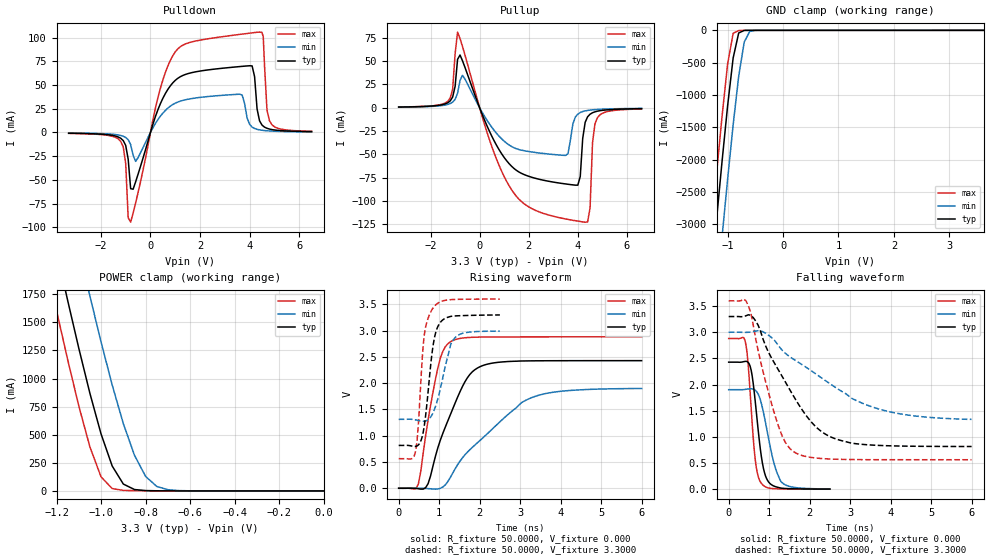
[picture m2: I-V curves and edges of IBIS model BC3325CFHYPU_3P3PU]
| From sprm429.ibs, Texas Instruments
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|   Model BC3325CFHYPU_3P3PU
[Model]   BC3325CFHYPU_3P3PU
Model_type   I/O
Polarity   Non-Inverting
Enable   Active-Low
Vinl =   0.9900V
Vinh =   2.3100V
Vmeas =   1.6500V
Cref =  15.0000pF
Rref = 100.0000M
Vref =  0.000V
C_comp   3.2113000062pf   3.3653001534pf   5.2276998132pf
[Temperature Range]   25.0000   0.1250k   -40.0000
[Voltage Range]   3.3000V   3.0000V   3.6000V
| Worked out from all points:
|   slope of the pulldown table from 0 to 0.495 V, typ, clamps not added: 13.9 ohm
|   slope of the pullup table from 0 to 0.495 V, typ, clamps not added: 16.3 ohm
|   GND clamp passes 1 mA (typ) near -0.67 V on its own axis
|   POWER clamp passes 1 mA (typ) near -0.73 V on its own axis
|   rising waveform, R_fixture 50.0000, V_fixture 0.000: 20-80 % time 712ps typ, 1.48ns min, 382ps max; typ from 0.001 V to 2.43 V
|   rising waveform, R_fixture 50.0000, V_fixture 3.3000: 20-80 % time 215ps typ, 312ps min, 166ps max; typ from 0.816 V to 3.3 V
|   falling waveform, R_fixture 50.0000, V_fixture 0.000: 20-80 % time 218ps typ, 319ps min, 166ps max; typ from 2.43 V to 0.003 V
|   falling waveform, R_fixture 50.0000, V_fixture 3.3000: 20-80 % time 1.13ns typ, 1.92ns min, 606ps max; typ from 3.3 V to 0.817 V
[Pulldown]
| voltage   I(typ)   I(min)   I(max)
-3.3V     -858uA     -614uA     -1.005mA
-1.2V     -6.162mA   -3.225mA   -9.462mA
-800mV    -59.28mA   -12.78mA   -94.65mA
-600mV    -52.16mA   -30.51mA   -74.44mA
1V        54.91mA    30.86mA    84.97mA
3.6V      69.44mA    40.27mA    103.4mA
4.1V      70.14mA    5.645mA    105mA
4.4V      12.22mA    2.696mA    105.8mA
4.55V     6.668mA    2.131mA    100.8mA
4.7V      4.353mA    1.744mA    23.59mA
4.8V      3.553mA    1.558mA    12.25mA
6.5V      840uA      548uA      1.176mA
|   6.6000   0.8040mA   0.5270mA   1.1160mA
[Pullup]
| voltage   I(typ)   I(min)   I(max)
-3.3V     805uA      687uA      859uA
-1.3V     5.391mA    3.609mA    6.959mA
-900mV    51.9mA     15.62mA    81.15mA
600mV     -35.88mA   -24.51mA   -49.07mA
1.7V      -70.21mA   -45.37mA   -100.4mA
3.5V      -81.59mA   -51.02mA   -119.1mA
4V        -82.9mA    -6.76mA    -121.4mA
4.3V      -15.54mA   -3.316mA   -122.6mA
4.5V      -6.855mA   -2.452mA   -107.1mA
4.6V      -5.294mA   -2.167mA   -37.4mA
4.8V      -3.613mA   -1.755mA   -10.57mA
6.6V      -914uA     -641uA     -1.25mA
[GND_clamp]
| voltage   I(typ)   I(min)   I(max)
-3.3V     -23.4A     -24.49A    -22.76A
-1.3V     -3.859A    -5.036A    -3.154A
-1.2V     -2.93A     -4.106A    -2.224A
-1.1V     -2.025A    -3.192A    -1.329A
-1V       -1.167A    -2.304A    -520.5mA
-900mV    -427.1mA   -1.461A    -46.43mA
-800mV    -40.98mA   -709.2mA   -2.872mA
-700mV    -1.416mA   -180.3mA   -459.5uA
-600mV    -185.8uA   -16.11mA   -224.9uA
-400mV    -135.4uA   -138.5uA   -210.3uA
3.62V     0A         0A         0A
[POWER_clamp]
| voltage   I(typ)   I(min)   I(max)
-3.3V     22.53A     23.34A     22.08A
-1.25V    2.586A     3.492A     2.054A
-1.2V     2.135A     3.04A      1.604A
-1.15V    1.695A     2.594A     1.168A
-1.05V    867.5mA    1.733A     390.4mA
-1V       506.6mA    1.325A     125mA
-950mV    221.5mA    942.3mA    21.03mA
-900mV    61.17mA    598.6mA    4.699mA
-850mV    12.39mA    317.4mA    2.279mA
-800mV    3.117mA    129.1mA    1.334mA
-750mV    1.236mA    39.97mA    732.8uA
0V        286.3pA    1.898nA    332.4pA
[Ramp]
| variable   typ   min   max
dV/dt_r   1.4399/0.6927n   0.7695/0.8573n   1.7265/0.3782n
dV/dt_f   1.3814/0.9941n   0.5983/0.9692n   1.8135/0.5956n
R_load = 50.0000
[Rising Waveform]
R_fixture = 50.0000
V_fixture = 0.000
V_fixture_min = 0.000
V_fixture_max = 0.000
| time   V(typ)   V(min)   V(max)
0s        1.182mV    1.135mV    1.272mV
484.8ps   -7.536mV   2.496mV    78.78mV
727.3ps   90.15mV    -4.991mV   1.301V
969.7ps   776.9mV    -12.18mV   2.298V
1.091ns   1.046V     25.6mV     2.607V
1.273ns   1.393V     201.9mV    2.784V
1.636ns   2.026V     636.8mV    2.863V
1.879ns   2.254V     821.1mV    2.874V
3.212ns   2.424V     1.701V     2.88V
6ns       2.428V     1.898V     2.88V
[Rising Waveform]
R_fixture = 50.0000
V_fixture = 3.3000
V_fixture_min = 3.0000
V_fixture_max = 3.6000
| time   V(typ)   V(min)   V(max)
0s        816mV      1.312V     564.1mV
404ps     796.5mV    1.303V     660.3mV
479.8ps   820.2mV    1.29V      1.147V
580.8ps   980.6mV    1.276V     2.462V
631.3ps   1.183V     1.276V     2.909V
833.3ps   2.626V     1.412V     3.411V
1.01ns    3.135V     1.831V     3.541V
1.288ns   3.27V      2.74V      3.588V
1.364ns   3.276V     2.839V     3.591V
2.5ns     3.297V     2.99V      3.599V
[Falling Waveform]
R_fixture = 50.0000
V_fixture = 0.000
V_fixture_min = 0.000
V_fixture_max = 0.000
| time   V(typ)   V(min)   V(max)
0s        2.428V     1.903V     2.88V
404ps     2.443V     1.907V     2.841V
479.8ps   2.426V     1.916V     2.398V
555.6ps   2.275V     1.919V     1.552V
656.6ps   1.675V     1.892V     563mV
808.1ps   621.6mV    1.638V     113mV
959.6ps   170.1mV    1.073V     30.1mV
1.111ns   63.19mV    521.9mV    12.27mV
1.288ns   22.97mV    151mV      7.218mV
2.5ns     3.182mV    6.45mV     1.833mV
[Falling Waveform]
R_fixture = 50.0000
V_fixture = 3.3000
V_fixture_min = 3.0000
V_fixture_max = 3.6000
| time   V(typ)   V(min)   V(max)
0s        3.3V       3V         3.6V
484.8ps   3.333V     2.999V     3.507V
727.3ps   3.135V     3.029V     2.649V
1.152ns   2.382V     2.826V     1.393V
1.394ns   2.058V     2.602V     904mV
1.636ns   1.735V     2.467V     702.9mV
2.182ns   1.173V     2.188V     594.7mV
2.788ns   928.6mV    1.872V     571.2mV
4ns       829.9mV    1.476V     564.6mV
6ns       816.8mV    1.335V     564.2mV
